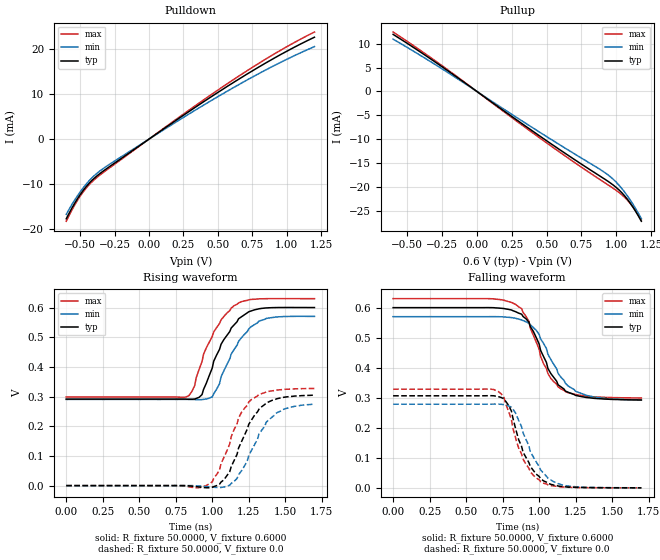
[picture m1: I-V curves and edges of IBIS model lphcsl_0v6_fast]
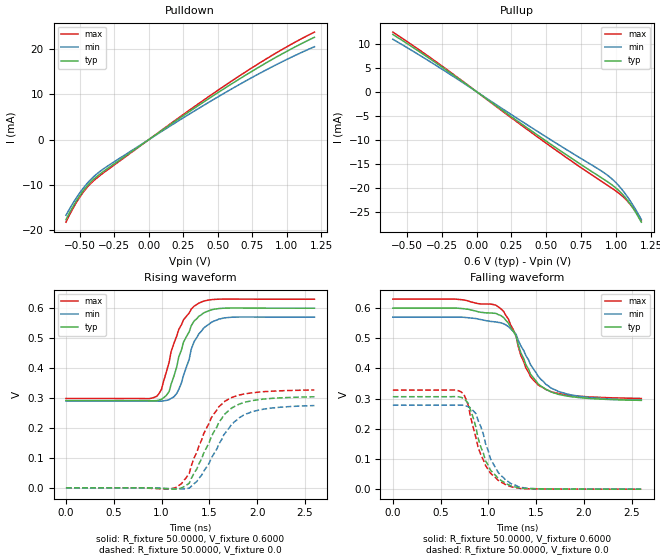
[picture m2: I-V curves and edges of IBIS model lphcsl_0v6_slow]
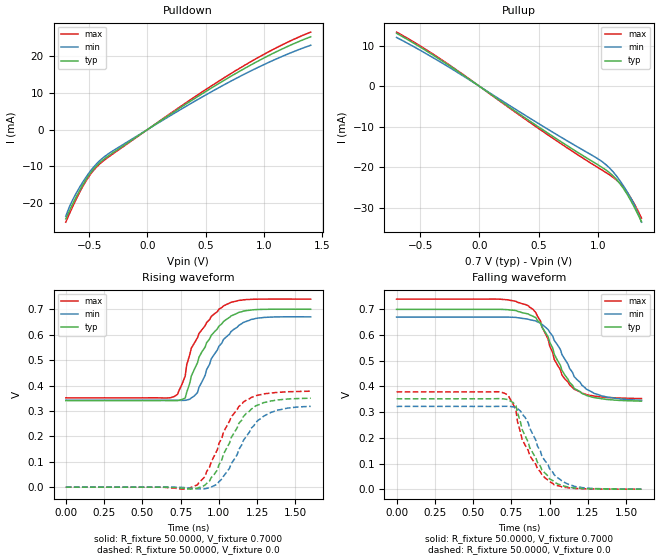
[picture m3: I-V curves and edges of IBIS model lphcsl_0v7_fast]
| Integrated Devices Technolgy, Inc
[IBIS Ver]   4.1
[File name]   9dbv0641.ibs
[File Rev]   1.5
|Rev history   1.5   include models for all settings, 21 July 2015
|Rev history   1.4   update LPRS_HCSL model , 09-23-2013
|Rev history   1.3   08-14 update IN data
|Rev history   1.2   08-14 update ^CKPWRGD_PD# data
|Rev history   1.1   08-13 update CLKIN data
|Rev history   1.0   original revision
[Date]   21 July 2015
[Disclaimer] Integrated Device Technology, Inc. ("IDT") hereby grants the
   user of this ibis model a non-exclusive, nontransferable
   license to use this ibis model under the following terms. the
   user is granted this license only to use the ibis model and is
   not granted rights to sell, copy (except as needed to run the
   ibis model), rent, lease or sub-license the ibis model in
   whole or in part, or in modified form to anyone. the user may
   modify the ibis model to suit its specific applications, but
   rights to derivative works and such modifications shall belong
   to idt. this ibis model is provided on an as is" basis and idt
   makes absolutely no warranty with respect to the information
   contained herein. idt disclaims and customer waives all
   warranties, express and implied, including warranties of
   merchantability and fitness for a particular purpose. the
   entire risk as to quality and performance is with the user
   accordingly, in no event shall idt be liable for any direct or
   indirect damages, whether in contract or tort, including any
   lost profits or other incidental, consequential, exemplary, or
   punitive damages arising out of the use or application of the
   ibis model. further, idt reserves the right to make changes
   without notice to any product herein to improve reliability,
   function, or design. idt does not convey any license under
   patent rights or any other intellectual property rights,
   including those of third parties. idt is not obligated to
   provide maintenance or support for the licensed ibis model.
[Copyright]   Copyright 2012, Integrated Devices Technolgy, Inc. all rights
   reserved
[Component]   9DBV0641
[Manufacturer] Integrated Device Technology, Inc.
[Package]
R_pkg   72.4655m   58.886m   86.045m
L_pkg   1.47175nH   1.11650nH   1.77850nH
C_pkg   0.07747pF   0.07444pF   0.08050pF
[Pin] signal_name  model_name
1 vSADR_tri   IN
2 ^vHIBW_BYPM_LOBW#   IN
3 FB_DNC   LPRS_HCSL
4 FB_DNC#   LPRS_HCSL
5 VDDR1.8   POWER
6 CLK_IN   CLKIN
7 CLK_IN#   CLKIN
8 GNDDIG   GND
9 SCLK_3.3   SCIN
10 SDATA_3.3   SCIN
11 VDDDIG1.8   POWER
12 VDDIO   POWER
13 vOE0#   IN
14 DIF0   LPRS_HCSL
15 DIF0#   LPRS_HCSL
16 VDD1.8   POWER
17 VDDIO   POWER
18 DIF1   LPRS_HCSL
19 DIF1#   LPRS_HCSL
20 NC   NC
21 vOE1#   IN
22 DIF2   LPRS_HCSL
23 DIF2#   LPRS_HCSL
24 vOE2#   IN
25 VDDA1.8   POWER
26 VDDIO   POWER
27 DIF3   LPRS_HCSL
28 DIF3#   LPRS_HCSL
29 vOE3#   IN
30 NC   NC
31 VDD1.8   POWER
32 VDDIO   POWER
33 DIF4   LPRS_HCSL
34 DIF4#   LPRS_HCSL
35 vOE4#   IN
36 DIF5   LPRS_HCSL
37 DIF5#   LPRS_HCSL
38 vOE5#   IN
39 VDDIO   POWER
40 ^CKPWRGD_PD#   PD
41 ePad   GND
[Diff Pin]  inv_pin  vdiff tdelay_typ tdelay_min  tdelay_max
3   4   NA   0   0   0
14   15   NA   0   0   0
18   19   NA   0   0   0
22   23   NA   0   0   0
27   28   NA   0   0   0
33   34   NA   0   0   0
36   37   NA   0   0   0
[Model Selector] LPRS_HCSL
lphcsl_0v6_fast amplitude 0.6V, slew rate fast
lphcsl_0v6_slow amplitude 0.6V, slew rate slow
lphcsl_0v7_fast amplitude 0.7V, slew rate fast
lphcsl_0v7_slow amplitude 0.7V, slew rate slow
lphcsl_0v8_fast amplitude 0.8V, slew rate fast
lphcsl_0v8_slow amplitude 0.8V, slew rate slow
lphcsl_0v9_fast amplitude 0.9V, slew rate fast
lphcsl_0v9_slow amplitude 0.9V, slew rate slow
| Models and submodels in the file (12): lphcsl_0v6_fast (Output), lphcsl_0v6_slow (Output), lphcsl_0v7_fast (Output), lphcsl_0v7_slow (Output), lphcsl_0v8_fast (Output), lphcsl_0v8_slow (Output), lphcsl_0v9_fast (Output), lphcsl_0v9_slow (Output), SCIN (Input), IN (Input), CLKIN (Input), PD (Input)
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[Model]   lphcsl_0v6_fast
Model_type Output
Polarity   Non-Inverting
Enable   Active-High
Vmeas =  0.4000V
Cref =   2.0000pF
Rref =   0.0
Vref =   0.4000V
C_comp   1.1000pF   1.0000pF   1.2000pF
[Temperature Range]   25.0000   75.0000   0.0
[Voltage Range]   0.6000V   0.5700V   0.6300V
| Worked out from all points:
|   slope of the pulldown table from 0 to 0.09 V, typ, clamps not added: 46.7 ohm
|   slope of the pullup table from 0 to 0.09 V, typ, clamps not added: 47.4 ohm
|   rising waveform, R_fixture 50.0000, V_fixture 0.6000: 20-80 % time 178ps typ, 179ps min, 178ps max; typ from 0.292 V to 0.6 V
|   rising waveform, R_fixture 50.0000, V_fixture 0.0: 20-80 % time 173ps typ, 176ps min, 168ps max; typ from 0 V to 0.305 V
|   falling waveform, R_fixture 50.0000, V_fixture 0.6000: 20-80 % time 182ps typ, 186ps min, 161ps max; typ from 0.6 V to 0.293 V
|   falling waveform, R_fixture 50.0000, V_fixture 0.0: 20-80 % time 140ps typ, 156ps min, 145ps max; typ from 0.306 V to 0 V
[Pulldown]
|Voltage   I(typ)   I(min)   I(max)
-600mV    -17.73mA   -16.75mA   -18.28mA
-540mV    -14.34mA   -13.62mA   -14.73mA
-480mV    -11.53mA   -10.95mA   -11.85mA
-440mV    -10.02mA   -9.465mA   -10.34mA
-400mV    -8.789mA   -8.218mA   -9.125mA
-320mV    -6.852mA   -6.295mA   -7.17mA
220mV     4.677mA    4.26mA     4.908mA
600mV     12.35mA    11.23mA    12.98mA
900mV     17.87mA    16.23mA    18.79mA
1.2V      22.67mA    20.58mA    23.82mA
[Pullup]
|Voltage   I(typ)   I(min)   I(max)
-600mV    11.94mA    10.94mA    12.43mA
-240mV    4.975mA    4.548mA    5.191mA
540mV     -11.13mA   -10.19mA   -11.61mA
940mV     -18.82mA   -17.47mA   -19.56mA
1V        -20.13mA   -19.02mA   -20.75mA
1.06V     -21.88mA   -21.09mA   -22.2mA
1.12V     -24.25mA   -23.65mA   -24.21mA
1.18V     -27.21mA   -26.66mA   -26.93mA
[Ramp]
| variable   typ   min   max
dV/dt_r  0.1828/0.1658n   0.1646/0.1750n   0.1965/0.1629n
dV/dt_f  0.1844/0.1738n   0.1666/0.1919n   0.1984/0.1620n
R_load = 50.0000
[Rising Waveform]
R_fixture= 50.0000
V_fixture= 0.6000
V_fixture_min= 0.5700
V_fixture_max= 0.6300
|time   V(typ)   V(min)   V(max)
0s        291.6mV    290.4mV    298.7mV
820ps     291.4mV    290.4mV    298.7mV
880ps     291.7mV    290.1mV    337.4mV
930ps     306.8mV    289.8mV    418.2mV
1ns       396.3mV    299.1mV    502.5mV
1.06ns    476mV      366.2mV    558.4mV
1.15ns    541.9mV    459.2mV    606.7mV
1.25ns    586mV      528.5mV    626.2mV
1.32ns    596mV      554.5mV    629.5mV
1.7ns     600.2mV    570.4mV    630.1mV
[Rising Waveform]
R_fixture= 50.0000
V_fixture= 0.0
V_fixture_min= 0.0
V_fixture_max= 0.0
|time   V(typ)   V(min)   V(max)
0s        0V         0V         0V
890ps     -3.58mV    -655.8uV   -7.526mV
1ns       -5.691mV   -4.788mV   12.59mV
1.05ns    4.772mV    -6.81mV    52.76mV
1.12ns    47.29mV    1.279mV    141.1mV
1.18ns    126.3mV    36.85mV    227.6mV
1.25ns    206.6mV    101.7mV    281.9mV
1.37ns    278.3mV    213.9mV    316.1mV
1.44ns    292.4mV    244.9mV    321.9mV
1.7ns     304.7mV    274.4mV    327.5mV
[Falling Waveform]
R_fixture= 50.0000
V_fixture= 0.6000
V_fixture_min= 0.5700
V_fixture_max= 0.6300
|time   V(typ)   V(min)   V(max)
0s        600mV      570mV      630mV
810ps     592.3mV    567mV      617.6mV
880ps     578.2mV    559.4mV    596.6mV
930ps     551.6mV    548.4mV    553.8mV
980ps     500.6mV    524.8mV    485.7mV
1.06ns    397.8mV    445.5mV    380.9mV
1.13ns    343.1mV    381.2mV    336.2mV
1.2ns     318mV      338.8mV    316.5mV
1.32ns    301.1mV    308.3mV    305.4mV
1.7ns     292.6mV    292.3mV    299.3mV
[Falling Waveform]
R_fixture= 50.0000
V_fixture= 0.0
V_fixture_min= 0.0
V_fixture_max= 0.0
|time   V(typ)   V(min)   V(max)
0s        306.5mV    278.5mV    328.5mV
690ps     306.6mV    278.8mV    327.3mV
760ps     296.2mV    277.1mV    300.6mV
810ps     256.1mV    268.7mV    227.7mV
820ps     233.2mV    262.8mV    199.6mV
890ps     118.8mV    182.7mV    95.62mV
1.01ns    30.83mV    59.83mV    20.86mV
1.06ns    15.44mV    32.63mV    10.17mV
1.18ns    3.389mV    7.484mV    2.238mV
1.7ns     139.5uV    252uV      103.6uV
[Model]   lphcsl_0v6_slow
Model_type Output
Polarity   Non-Inverting
Enable   Active-High
Vmeas =  0.4000V
Cref =   2.0000pF
Rref =   0.0
Vref =   0.4000V
C_comp   1.1000pF   1.0000pF   1.2000pF
[Temperature Range]   25.0000   75.0000   0.0
[Voltage Range]   0.6000V   0.5700V   0.6300V
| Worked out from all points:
|   slope of the pulldown table from 0 to 0.09 V, typ, clamps not added: 46.7 ohm
|   slope of the pullup table from 0 to 0.09 V, typ, clamps not added: 47.4 ohm
|   rising waveform, R_fixture 50.0000, V_fixture 0.6000: 20-80 % time 199ps typ, 187ps min, 207ps max; typ from 0.292 V to 0.6 V
|   rising waveform, R_fixture 50.0000, V_fixture 0.0: 20-80 % time 287ps typ, 320ps min, 278ps max; typ from 0 V to 0.304 V
|   falling waveform, R_fixture 50.0000, V_fixture 0.6000: 20-80 % time 277ps typ, 310ps min, 249ps max; typ from 0.6 V to 0.294 V
|   falling waveform, R_fixture 50.0000, V_fixture 0.0: 20-80 % time 196ps typ, 203ps min, 199ps max; typ from 0.306 V to 0 V
[Pulldown]
|Voltage   I(typ)   I(min)   I(max)
-600mV    -17.73mA   -16.75mA   -18.28mA
-540mV    -14.34mA   -13.62mA   -14.73mA
-480mV    -11.53mA   -10.95mA   -11.85mA
-440mV    -10.02mA   -9.465mA   -10.34mA
-400mV    -8.789mA   -8.218mA   -9.125mA
-320mV    -6.852mA   -6.295mA   -7.17mA
220mV     4.677mA    4.26mA     4.908mA
600mV     12.35mA    11.23mA    12.98mA
900mV     17.87mA    16.23mA    18.79mA
1.2V      22.67mA    20.58mA    23.82mA
[Pullup]
|Voltage   I(typ)   I(min)   I(max)
-600mV    11.94mA    10.94mA    12.43mA
-240mV    4.975mA    4.548mA    5.191mA
540mV     -11.13mA   -10.19mA   -11.61mA
940mV     -18.82mA   -17.47mA   -19.56mA
1V        -20.13mA   -19.02mA   -20.75mA
1.06V     -21.88mA   -21.09mA   -22.2mA
1.12V     -24.25mA   -23.65mA   -24.21mA
1.18V     -27.21mA   -26.66mA   -26.93mA
[Ramp]
| variable   typ   min   max
dV/dt_r  0.1826/0.2924n   0.1649/0.3119n   0.1961/0.2863n
dV/dt_f  0.1834/0.2952n   0.1651/0.3356n   0.1975/0.2766n
R_load = 50.0000
[Rising Waveform]
R_fixture= 50.0000
V_fixture= 0.6000
V_fixture_min= 0.5700
V_fixture_max= 0.6300
|time   V(typ)   V(min)   V(max)
0s        291.6mV    290.4mV    298.7mV
950ps     291.5mV    290mV      306.1mV
1ns       295.8mV    289.9mV    329.4mV
1.08ns    322.2mV    294.9mV    420.6mV
1.16ns    405.4mV    315.9mV    508.1mV
1.23ns    486.8mV    376mV      561.2mV
1.31ns    541mV      461.9mV    596.7mV
1.44ns    584.4mV    533.5mV    623.7mV
1.68ns    600.4mV    568.5mV    630.7mV
2.6ns     600.1mV    570.2mV    630.1mV
[Rising Waveform]
R_fixture= 50.0000
V_fixture= 0.0
V_fixture_min= 0.0
V_fixture_max= 0.0
|time   V(typ)   V(min)   V(max)
0s        0V         0V         0V
1.16ns    -3.564mV   -2.85mV    2.387mV
1.29ns    15.53mV    -1.023mV   47.73mV
1.34ns    48.97mV    13.95mV    99.71mV
1.37ns    63.74mV    21.58mV    119mV
1.52ns    170.6mV    99.09mV    233.8mV
1.65ns    243mV      176.5mV    286.9mV
1.81ns    279.5mV    233.7mV    310mV
1.94ns    291.2mV    253.8mV    317.4mV
2.6ns     304.3mV    274.9mV    326.9mV
[Falling Waveform]
R_fixture= 50.0000
V_fixture= 0.6000
V_fixture_min= 0.5700
V_fixture_max= 0.6300
|time   V(typ)   V(min)   V(max)
0s        600mV      570mV      630mV
1.08ns    582.5mV    554.3mV    609.7mV
1.16ns    568.6mV    548.2mV    589mV
1.29ns    507.2mV    513.2mV    507.8mV
1.34ns    451.9mV    474.6mV    442.6mV
1.39ns    413.8mV    444.1mV    403.1mV
1.52ns    349.3mV    374.6mV    345.2mV
1.65ns    323mV      336.1mV    323.8mV
1.86ns    306.7mV    312.7mV    310.9mV
2.6ns     294.4mV    294.9mV    300.8mV
[Falling Waveform]
R_fixture= 50.0000
V_fixture= 0.0
V_fixture_min= 0.0
V_fixture_max= 0.0
|time   V(typ)   V(min)   V(max)
0s        306.5mV    278.5mV    328.5mV
740ps     301.4mV    278.3mV    316.4mV
790ps     283.8mV    273.5mV    277.5mV
870ps     204.4mV    250.2mV    169.9mV
970ps     93.57mV    151.3mV    78.02mV
1.02ns    63.97mV    102.1mV    53.95mV
1.1ns     36.32mV    56.87mV    29.84mV
1.21ns    14.87mV    24.69mV    11.18mV
1.44ns    1.542mV    2.554mV    1.221mV
2.6ns     153.2uV    211.3uV    128.1uV
[Model]   lphcsl_0v7_fast
Model_type Output
Polarity   Non-Inverting
Enable   Active-High
Vmeas =  0.4000V
Cref =   2.0000pF
Rref =   0.0
Vref =   0.4000V
C_comp   1.1000pF   1.0000pF   1.2000pF
[Temperature Range]   25.0000   75.0000   0.0
[Voltage Range]   0.7000V   0.6700V   0.7400V
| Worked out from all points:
|   slope of the pulldown table from 0 to 0.105 V, typ, clamps not added: 46.7 ohm
|   slope of the pullup table from 0 to 0.105 V, typ, clamps not added: 48.9 ohm
|   rising waveform, R_fixture 50.0000, V_fixture 0.7000: 20-80 % time 184ps typ, 189ps min, 167ps max; typ from 0.341 V to 0.7 V
|   rising waveform, R_fixture 50.0000, V_fixture 0.0: 20-80 % time 172ps typ, 185ps min, 179ps max; typ from 0 V to 0.35 V
|   falling waveform, R_fixture 50.0000, V_fixture 0.7000: 20-80 % time 180ps typ, 197ps min, 166ps max; typ from 0.7 V to 0.343 V
|   falling waveform, R_fixture 50.0000, V_fixture 0.0: 20-80 % time 157ps typ, 161ps min, 146ps max; typ from 0.352 V to 0 V
[Pulldown]
|Voltage   I(typ)   I(min)   I(max)
-700mV    -24.35mA   -23.64mA   -25.28mA
-670mV    -22.26mA   -21.16mA   -23.07mA
-640mV    -20.25mA   -19.13mA   -20.95mA
-580mV    -16.55mA   -15.66mA   -17.03mA
-520mV    -13.34mA   -12.68mA   -13.69mA
-430mV    -9.691mA   -9.131mA   -10.02mA
-340mV    -7.298mA   -6.726mA   -7.628mA
230mV     4.886mA    4.45mA     5.127mA
680mV     13.88mA    12.62mA    14.59mA
1.04V     20.22mA    18.36mA    21.25mA
1.22V     22.96mA    20.85mA    24.13mA
1.4V      25.34mA    23.03mA    26.62mA
[Pullup]
|Voltage   I(typ)   I(min)   I(max)
-700mV    13.05mA    12.03mA    13.35mA
-490mV    9.468mA    8.696mA    9.752mA
-310mV    6.146mA    5.633mA    6.355mA
500mV     -10.03mA   -9.194mA   -10.4mA
800mV     -15.73mA   -14.45mA   -16.3mA
1.04V     -20.06mA   -18.64mA   -20.72mA
1.13V     -22.08mA   -21.08mA   -22.44mA
1.22V     -25.3mA    -24.66mA   -24.97mA
1.25V     -26.68mA   -26.08mA   -26.14mA
1.31V     -29.84mA   -29.28mA   -29.02mA
1.34V     -31.57mA   -31.17mA   -30.68mA
1.37V     -33.4mA    -33.5mA    -32.47mA
[Ramp]
| variable   typ   min   max
dV/dt_r  0.2101/0.1771n   0.1909/0.1879n   0.2266/0.1755n
dV/dt_f  0.2143/0.1763n   0.1943/0.1928n   0.2323/0.1650n
R_load = 50.0000
[Rising Waveform]
R_fixture= 50.0000
V_fixture= 0.7000
V_fixture_min= 0.6700
V_fixture_max= 0.7400
|time   V(typ)   V(min)   V(max)
0s        340.9mV    342mV      351.5mV
710ps     340.3mV    342mV      357.1mV
780ps     350.7mV    341.7mV    436.8mV
790ps     373.5mV    343.1mV    481.7mV
820ps     437.2mV    351.1mV    546.8mV
860ps     489mV      371.9mV    587.6mV
950ps     597.2mV    505.1mV    671.9mV
1.03ns    651.8mV    581.1mV    713.2mV
1.21ns    697.1mV    659.9mV    739.1mV
1.6ns     700.1mV    670.3mV    740.1mV
[Rising Waveform]
R_fixture= 50.0000
V_fixture= 0.0
V_fixture_min= 0.0
V_fixture_max= 0.0
|time   V(typ)   V(min)   V(max)
0s        0V         0V         0V
810ps     -7.521mV   -3.728mV   -3.151mV
910ps     8.285mV    -6.321mV   42.33mV
990ps     67.83mV    11.68mV    147.1mV
1.03ns    130.4mV    42.94mV    216.4mV
1.08ns    194.2mV    91.72mV    275.7mV
1.16ns    277.7mV    184mV      335mV
1.24ns    320mV      253.8mV    360.2mV
1.31ns    334.7mV    285mV      368.4mV
1.6ns     350.1mV    318.1mV    377.6mV
[Falling Waveform]
R_fixture= 50.0000
V_fixture= 0.7000
V_fixture_min= 0.6700
V_fixture_max= 0.7400
|time   V(typ)   V(min)   V(max)
0s        700mV      670mV      740mV
680ps     700mV      670.1mV    739.5mV
840ps     684.7mV    663.5mV    719.1mV
910ps     667.5mV    654.9mV    687.2mV
990ps     593.6mV    621.5mV    584.4mV
1.03ns    525.9mV    579.3mV    505.2mV
1.08ns    463.2mV    524.7mV    445mV
1.16ns    392.3mV    438.1mV    389.5mV
1.29ns    356.6mV    373mV      362.4mV
1.6ns     342.9mV    346.1mV    352.9mV
[Falling Waveform]
R_fixture= 50.0000
V_fixture= 0.0
V_fixture_min= 0.0
V_fixture_max= 0.0
|time   V(typ)   V(min)   V(max)
0s        351.9mV    322.2mV    378.7mV
710ps     350.9mV    322.7mV    372.3mV
780ps     325.6mV    318.9mV    307.6mV
790ps     297.8mV    313.5mV    262.9mV
820ps     232.9mV    292.8mV    194.6mV
840ps     207.9mV    279.3mV    171.4mV
920ps     104.8mV    168.4mV    80.17mV
1ns       40.1mV     79.05mV    29.21mV
1.16ns    4.805mV    11.18mV    3.196mV
1.6ns     236.9uV    414.6uV    176.6uV
